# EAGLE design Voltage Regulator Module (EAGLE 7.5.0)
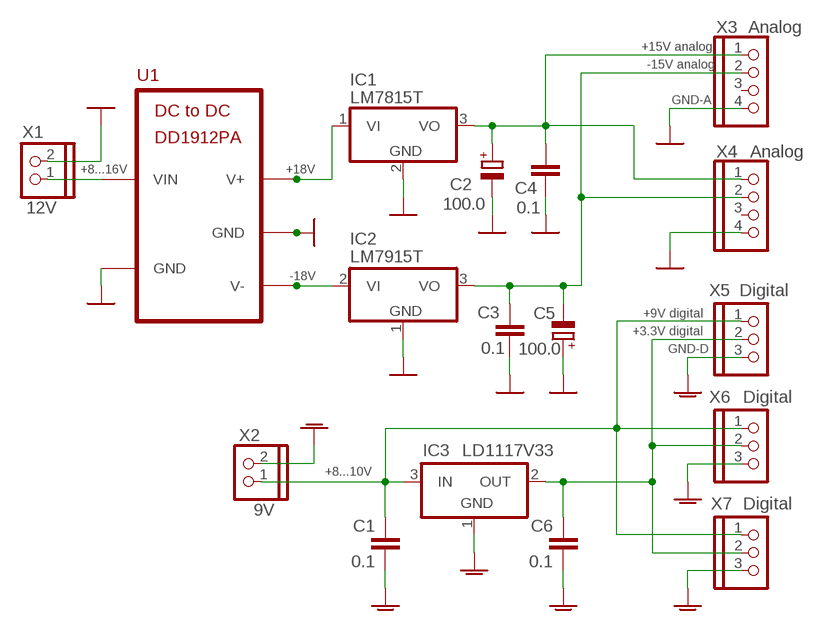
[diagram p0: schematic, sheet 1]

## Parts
C1  0.1  C-EU050-025X075  [C050-025X075]
C2  100.0  CPOL-EUE2.5-6  [E2,5-6]
C3  0.1  C-EU050-025X075  [C050-025X075]
C4  0.1  C-EU050-025X075  [C050-025X075]
C5  100.0  CPOL-EUE2.5-6  [E2,5-6]
C6  0.1  C-EU050-025X075  [C050-025X075]
IC1  LM7815T  7815TV  [TO220V]
IC2  LM7915T  7912VT  [7912-VERT]
IC3  LD1117V33  LM1117V-3.3_IN_TO-220  [LM1117-VERT]
U1  BIPOLAR-POWER-MODULE-DD1912PA  [5-PIN-MODULE-DD1912PA]
X1  12V  PINHD-1X2  [1X02]
X2  9V  PINHD-1X2  [1X02]
X3  Analog  PINHD-1X4  [1X04]
X4  Analog  PINHD-1X4  [1X04]
X5  Digital  PINHD-1X3  [1X03]
X6  Digital  PINHD-1X3  [1X03]
X7  Digital  PINHD-1X3  [1X03]

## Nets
3V3-D: C6.2 IC3.2(OUT) X5.2 X6.2 X7.2
9V-D: C1.2 IC3.3(IN) X2.1 X5.1 X6.1 X7.1
+15V-A: C2.+ C4.2 IC1.3(VO) X3.1 X4.1
-15V-A: C3.2 C5.- IC2.3(VO) X3.2 X4.2
GND-A: C2.- C3.1 C4.1 C5.+ IC1.2(GND) IC2.1(GND) U1.IN.2(GND) U1.OUT.2(GND) X1.2 X3.4 X4.4 ; supply symbol labelled GND
GND-D: C1.1 C6.1 IC3.1(GND) X2.2 X5.3 X6.3 X7.3 ; supply symbol labelled GNDA
V+: IC1.1(VI) U1.OUT.3(V+)
V-: IC2.2(VI) U1.OUT.1(V-)
VIN: U1.IN.1(VIN) X1.1
Unconnected: X3.3 X4.3

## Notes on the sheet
- +15V analog
- -15V analog
- GND-A
- +8...16V | +18V
- -18V
- +9V digital
- +3.3V digital
- GND-D
- +8...10V

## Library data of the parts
C1 C3 C4 C6 = rcl:C-EU: CAPACITOR, European symbol
C2 C5 = rcl:CPOL-EU: POLARIZED CAPACITOR, European symbol
IC1 = linear:78*: Positive VOLTAGE REGULATOR Source: http://cache.national.com/ds/LM/LM78L05.pdf http://www.fairchildsemi.com/ds/LM/LM7805.pdf
IC2 = FRMeterCustomComponents:7912VT
IC3 = FRMeterCustomComponents:LM1117V-3.3_IN_TO-220
U1 = FRMeterCustomComponents:BIPOLAR-POWER-MODULE-DD1912PA: DC-DC converter +9V to +/-15V
X1 X2 = pinhead:PINHD-1X2: PIN HEADER
X3 X4 = pinhead:PINHD-1X4: PIN HEADER
X5-X7 = pinhead:PINHD-1X3: PIN HEADER

## Module ISOLATED_CONVERTER
Ports: IN-(nc) OUT-(nc) OUT+(nc) IN+(nc)

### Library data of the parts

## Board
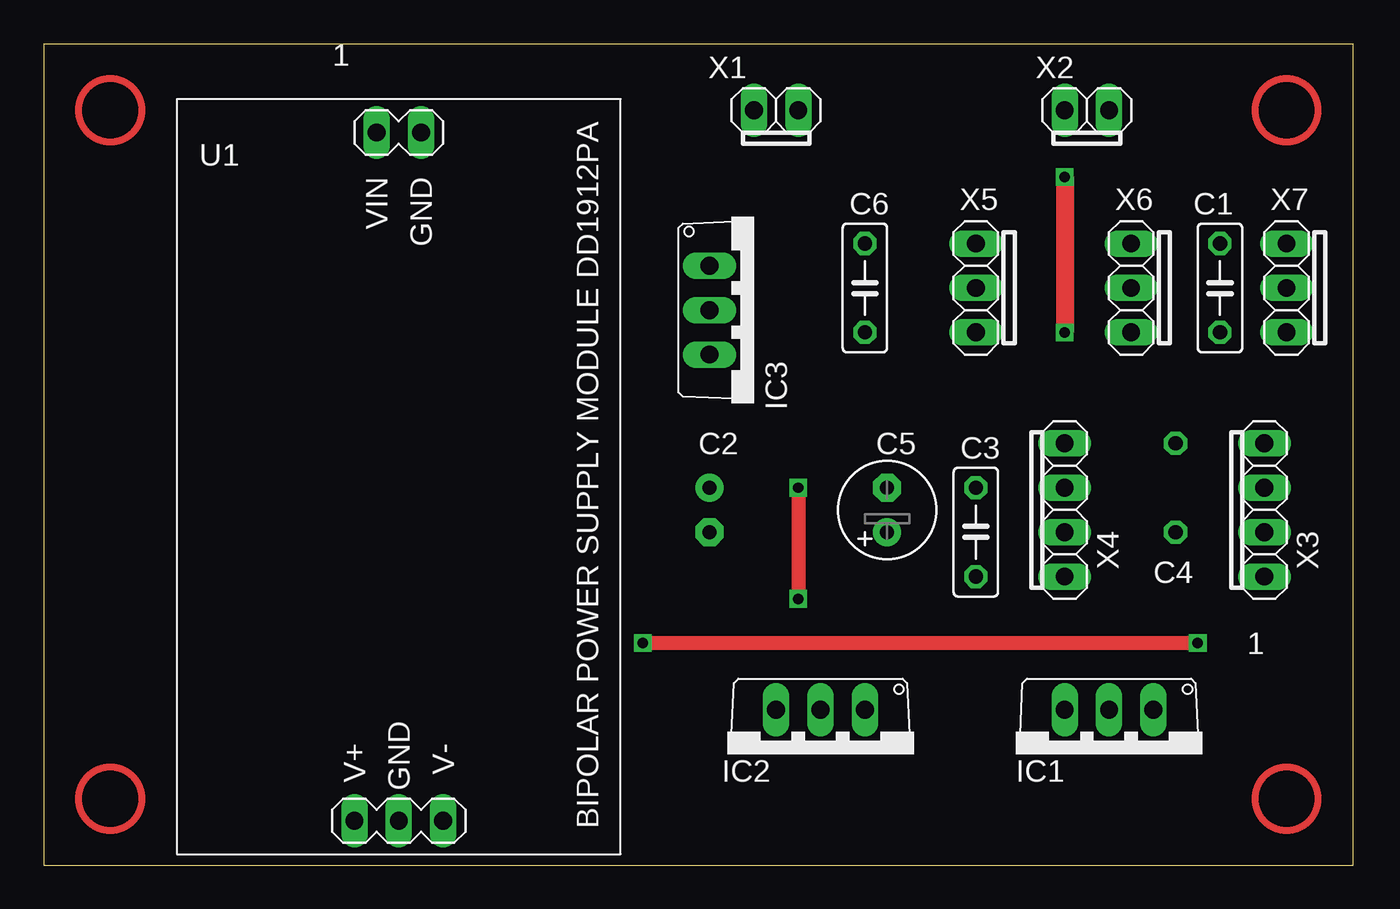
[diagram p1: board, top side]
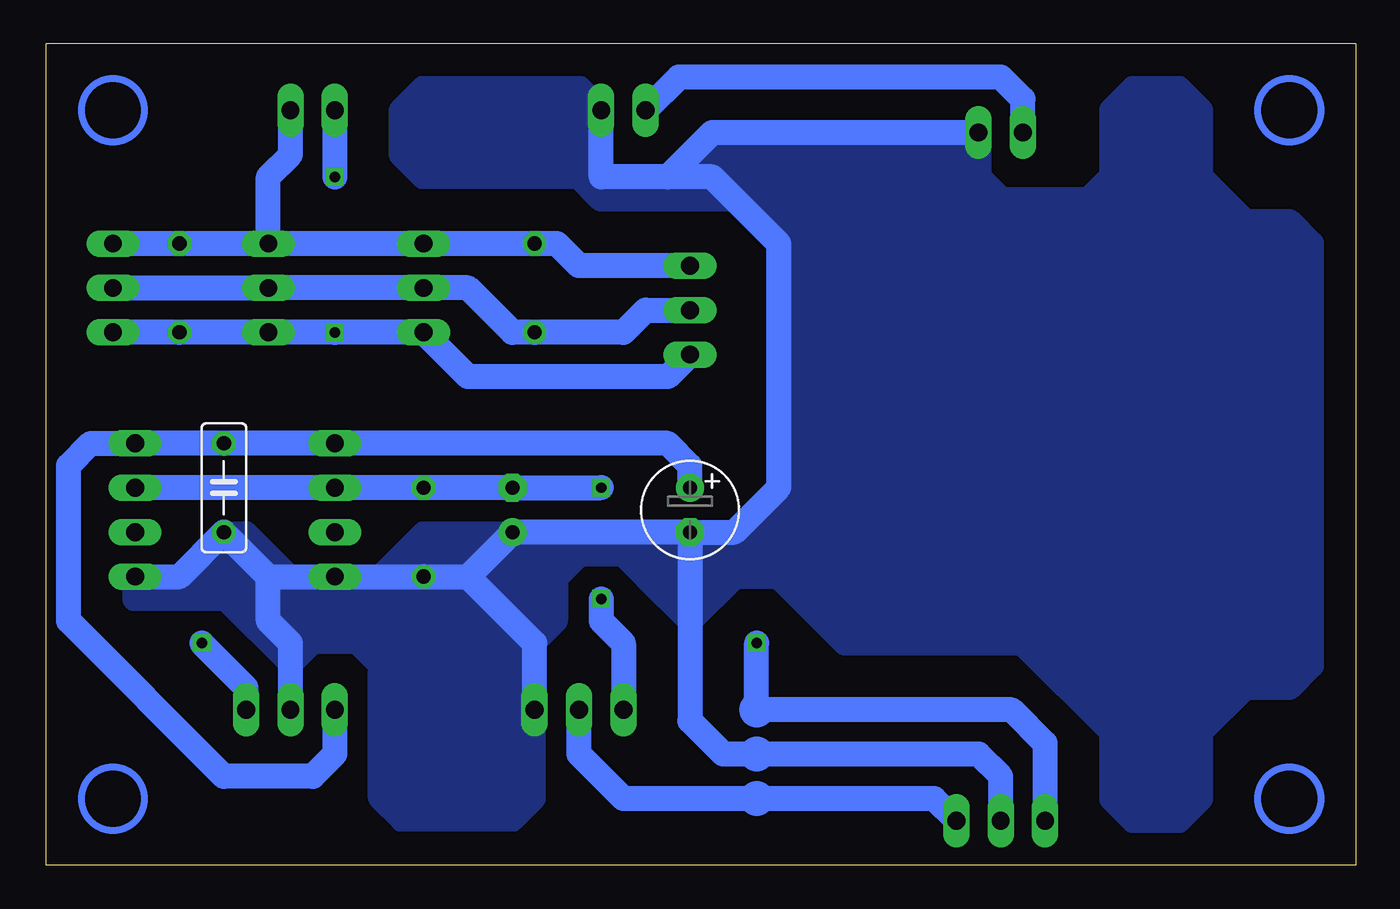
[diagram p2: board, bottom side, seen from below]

Size 74.93 x 46.99 mm. Coordinates in mm from the lower left corner, seen from the top.
Outline: 0,0 74.93,0 74.93,46.99 0,46.99 0,0
Copper layers (1*16): Top 0.035mm / dielectric 1.5mm / Bottom 0.035mm
Design rules "default *": minimum track width 10mil, minimum drill 4mil, track to track 8mil, track to pad 8mil, pad to pad 8mil, via to via 8mil, smd to smd 8mil, copper to edge 0mil, drill to drill 8mil, minimum pad ring 10mil, minimum via ring 8mil, stop-mask expansion 4mil, vias tented up to drill 0mil, thermal gap 10mil

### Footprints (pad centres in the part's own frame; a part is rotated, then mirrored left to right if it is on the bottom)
C050-025X075 = drill 0.813 octagon: 1 -2.54,0; 2 2.54,0
E2,5-6 = drill 0.813 pad 1.6: + -1.27,0 | drill 0.813 pad 1.6 octagon: - 1.27,0
TO220V = drill 1.016 long: 1 -2.54,-2.54; 2 0,-2.54; 3 2.54,-2.54
7912-VERT = drill 1.016 long: 1 -2.54,0; 2 0,0; 3 2.54,0
LM1117-VERT = drill 1.016 long: 1 -2.54,0; 2 0,0; 3 2.54,0
5-PIN-MODULE-DD1912PA = drill 1.016 long: IN.1 -19.685,-1.27; IN.2 -19.685,1.27; OUT.1 19.685,2.54; OUT.2 19.685,0; OUT.3 19.685,-2.54
1X02 = drill 1.016 long: 1 -1.27,0; 2 1.27,0
1X04 = drill 1.016 long: 1 -3.81,0; 2 -1.27,0; 3 1.27,0; 4 3.81,0
1X03 = drill 1.016 long: 1 -2.54,0; 2 0,0; 3 2.54,0

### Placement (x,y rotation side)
C1  67.31,33.02 270 top
C2  38.1,20.32 270 bottom
C3  53.34,19.05 90 top
C4  64.77,21.59 90 bottom
C5  48.26,20.32 90 top
C6  46.99,33.02 270 top
IC1  60.96,6.35 180 top
IC2  44.45,8.89 180 top
IC3  38.1,31.75 270 top
U1  20.32,22.22 270 top
X1  41.91,43.18 0 top
X2  59.69,43.18 0 top
X3  69.85,20.32 270 top
X4  58.42,20.32 270 top
X5  53.34,33.02 90 top
X6  62.23,33.02 90 top
X7  71.12,33.02 90 top

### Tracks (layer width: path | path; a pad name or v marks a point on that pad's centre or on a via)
3V3-D
  Bottom 1.422: X7.2 X6.2 X5.2 50.8,33.02 48.26,30.48 C6.2 41.91,30.48 40.64,31.75 IC3.2
9V-D  (via drill 0.6)
  Top 1.016: v58.42,39.37 v58.42,30.48
  Bottom 1.422: IC3.3 39.37,27.94 50.8,27.94 X5.1 v58.42,30.48 X6.1 C1.2 X7.1 | X2.1 v58.42,39.37
+15V-A
  Bottom 1.422: C2.+ 38.1,22.86 39.37,24.13 X4.1 C4.2 X3.1 72.39,24.13 73.66,22.86 73.66,13.97 64.77,5.08 59.69,5.08 58.42,6.35 IC1.3
-15V-A  (via drill 0.6)
  Top 0.813: v43.18,21.59 v43.18,15.24
  Bottom 1.422: X3.2 X4.2 C3.2 C5.- v43.18,21.59 | v43.18,15.24 43.18,13.97 41.91,12.7 IC2.3
GND-A
  Bottom 1.422: X3.4 67.31,16.51 C4.1 62.23,16.51 | 62.23,16.51 X4.4 C3.1 50.8,16.51 | IC2.1 46.99,12.7 50.8,16.51 | U1.OUT.2 20.32,5.08 21.59,6.35 36.2,6.35 38.1,8.25 C2.- | C2.- C5.+ 50.8,16.51 | IC1.2 60.96,12.7 62.23,13.97 62.23,16.51 | U1.IN.2 36.83,41.91 39.37,39.37 | 39.37,39.37 43.18,39.37 X1.2 | C2.- 35.56,19.05 33.02,21.59 33.02,35.56 36.83,39.37 39.37,39.37
  pour Bottom (no thermals): 46.99,12.7 46.99,3.81 48.26,2.54 54.61,2.54 55.88,3.81 55.88,11.43 57.15,12.7 59.69,12.7 60.96,11.43 64.77,15.24 66.04,15.24 67.31,16.51 64.77,19.05 63.5,19.05 60.96,16.51 55.88,16.51 53.34,19.05 44.45,19.05 45.72,17.78 45.72,13.97
  pour Bottom (no thermals): 38.1,13.97 40.64,16.51 40.64,17.78 41.91,19.05 35.56,19.05 33.02,21.59 33.02,35.56 36.83,39.37 39.37,39.37 36.83,41.91 21.59,41.91 21.59,39.37 20.32,38.1 15.24,38.1 13.97,39.37 13.97,43.18 12.7,44.45 10.16,44.45 8.89,43.18 8.89,39.37 6.35,36.83 3.81,36.83 2.54,35.56 2.54,11.43 3.81,10.16 6.35,10.16 8.89,7.62 8.89,3.81 10.16,2.54 12.7,2.54 13.97,3.81 13.97,7.62 19.05,12.7 29.21,12.7 33.02,16.51 35.56,16.51
  pour Bottom (no thermals): 39.37,19.05 39.37,15.24 41.91,17.78 44.45,17.78 46.99,15.24 46.99,19.05
  pour Bottom (no thermals): 69.85,16.51 63.5,16.51 63.5,15.24 69.85,15.24
  pour Bottom (no thermals): 43.18,39.37 34.29,39.37 34.29,38.1 43.18,38.1 44.45,39.37 53.34,39.37 54.61,40.64 54.61,43.18 53.34,44.45 44.45,44.45 43.18,43.18
GND-D
  Bottom 1.422: IC3.1 44.45,34.29 45.72,35.56 C6.1 X5.3 X6.3 | X6.3 C1.1 X7.3 | X6.3 62.23,39.37 60.96,40.64 X2.2
V+  (via drill 0.6)
  Top 0.813: v66.04,12.7 v34.29,12.7
  Bottom 1.422: IC1.1 63.5,10.16 v66.04,12.7 | U1.OUT.3 17.78,6.99 19.69,8.89 34.29,8.89 v34.29,12.7
V-
  Bottom 1.422: U1.OUT.1 24.13,3.81 41.91,3.81 44.45,6.35 IC2.2
VIN
  Bottom 1.422: U1.IN.1 19.05,43.82 20.32,45.09 38.73,45.09 X1.1
(copper drawn outside any net)
  shapes: Bottom circle x7, Top circle x4

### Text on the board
tPlace: 1 | 1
